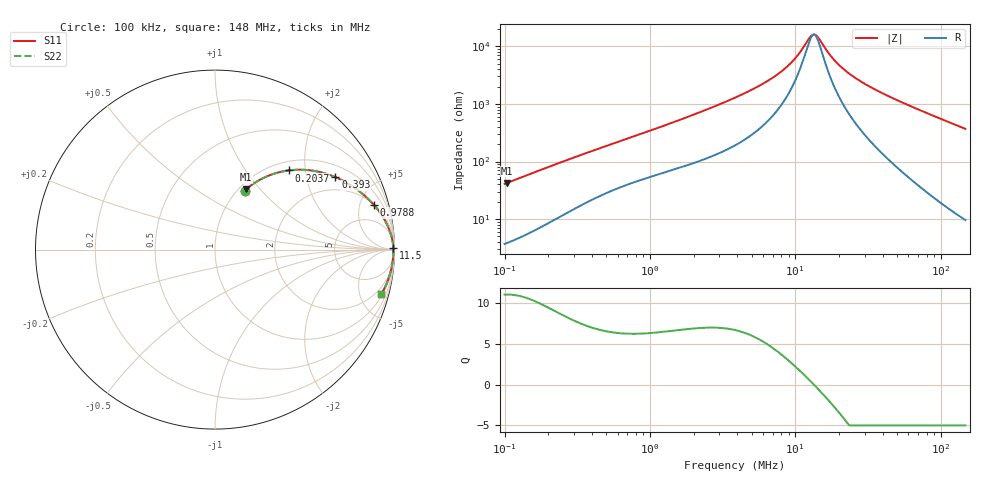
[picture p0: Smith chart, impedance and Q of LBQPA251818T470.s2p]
! LBQPA251818T470  S-PARAMETER MODEL  ( General Type )
! Model Generated by TAIYO YUDEN Corporation (http://www.ty-top.com)
! Version 1.0
! TAIYO YUDEN Control No. 191025NI43SB-FBB
! Copyright(c) 2019 TAIYO YUDEN CO.,LTD. All Rights Reserved.
! Product Description (link to TY-COMPAS)
! https://ds.yuden.co.jp/TYCOMPAS/or/detail?pn=LBQPA251818T470K&u=M
! Products Name : Inductors
! Characteristics :
!  Inductance : 47 uH , SRF(min) : 12 MHz , DC Resistance(max) : 2.47 Ohm
!  Rated Current : Saturation :240 mA , Temp Rise : 165 mA (20 degC)
!  Case Size : 2.5 x 1.8 / 0.098 x 0.071 [mm/inch] , Thickness : 1.8 / 0.071 [mm/inch]
!  (Conditions: Temperature = 25 degC , DC Bias Current/Voltage = 0A / 0V)
! External Node Assignments :
!  1  o---GGG---o  2
! GND o---------o GND
! Frequency Range : 0.1MHz  -  147.97148MHz  [ 402 STEP ]
# MHz S RI R 50
! Freq[MHz].  S11 Real  S11 Imag  S21 Real  S21 Imag  S12 Real  S12 Imag  S22 Real  S22 Imag
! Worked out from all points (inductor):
!   401 points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, 100 kHz to 148 MHz, reference 50 ohm
!   read as one part in series: L = 64.6 uH near 103.7 kHz
!   highest Q = 11 at 103.7 kHz (marker M1), where L = 64.8 uH
!   self-resonance near 13.31 MHz
!   S11 on the Smith chart (normalised r, x): 100 kHz: 1.07, +0.82; 203.7 kHz: 1.17, +1.63; 393 kHz: 1.43, +2.97; 978.8 kHz: 2.06, +6.64; 11.5 MHz: open; 148 MHz: 1.19, -7.39
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0.1  0.1648 0.3283  0.8352 -0.3283  0.8352 -0.3283  0.1648 0.3283
0.103717  0.1738 0.3362  0.8262 -0.3362  0.8262 -0.3362  0.1738 0.3362
0.203748  0.4101 0.4411  0.5899 -0.4411  0.5899 -0.4411  0.4101 0.4411
0.339629  0.6188 0.4228  0.3812 -0.4228  0.3812 -0.4228  0.6188 0.4228
0.393014  0.6706 0.4039  0.3294 -0.4039  0.3294 -0.4039  0.6706 0.4039
0.609002  0.7954 0.3317  0.2046 -0.3317  0.2046 -0.3317  0.7954 0.3317
0.97877  0.8855 0.2486  0.1145 -0.2486  0.1145 -0.2486  0.8855 0.2486
1.153479  0.9079 0.2214  0.0921 -0.2214  0.0921 -0.2214  0.9079 0.2214
3.917549  0.9833 0.0733  0.0167 -0.0733  0.0167 -0.0733  0.9833 0.0733
5.747101  0.9894 0.0456  0.0106 -0.0456  0.0106 -0.0456  0.9894 0.0456
7.695838  0.9919 0.0282  0.00806 -0.0282  0.00806 -0.0282  0.9919 0.0282
9.579906  0.993 0.0166  0.00697 -0.0166  0.00697 -0.0166  0.993 0.0166
11.49783  0.9936 0.00751  0.00642 -0.00751  0.00642 -0.00751  0.9936 0.00751
13.06453  0.9938 0.00126  0.0062 -0.00126  0.0062 -0.00126  0.9938 0.00126
13.55017  0.9938 -0.000513  0.00616 0.000513  0.00616 0.000513  0.9938 -0.000513
14.31268  0.9939 -0.00318  0.00612 0.00318  0.00612 0.00318  0.9939 -0.00318
18.14478  0.9938 -0.015  0.00615 0.015  0.00615 0.015  0.9938 -0.015
22.58693  0.9935 -0.0266  0.00654 0.0266  0.00654 0.0266  0.9935 -0.0266
30.24575  0.9923 -0.0442  0.00773 0.0442  0.00773 0.0442  0.9923 -0.0442
44.37094  0.9888 -0.0731  0.0112 0.0731  0.0112 0.0731  0.9888 -0.0731
82.52087  0.9729 -0.1432  0.0271 0.1432  0.0271 0.1432  0.9729 -0.1432
147.9715  0.9261 -0.2489  0.0739 0.2489  0.0739 0.2489  0.9261 -0.2489
